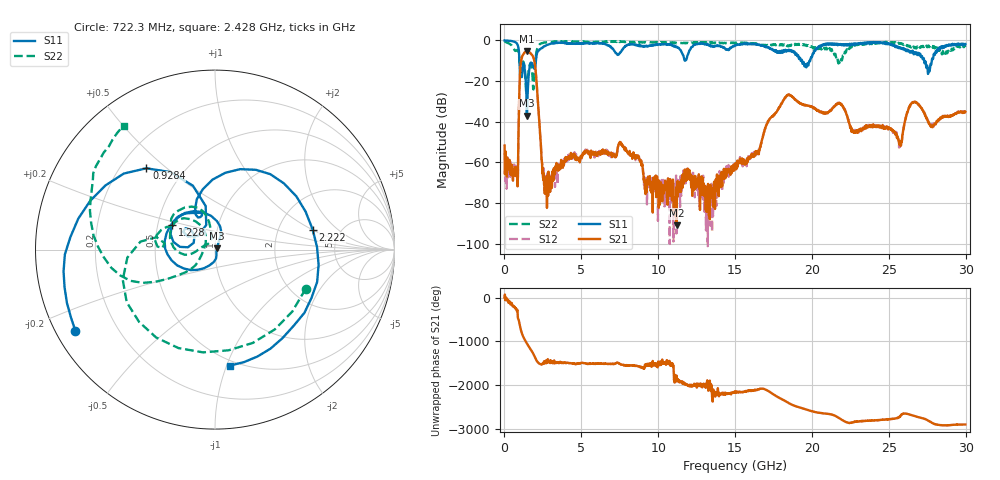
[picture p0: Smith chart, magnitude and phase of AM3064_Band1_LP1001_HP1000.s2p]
# Hz S DB R 50.0
!freq dBS11 angS11 dBS21 angS21 dBS12 angS12 dBS22 angS22
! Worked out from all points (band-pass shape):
!   1600 points, 10 MHz to 29.98 GHz, reference 50 ohm
!   highest |S21| = -5.26 dB at 1.472 GHz (marker M1); lowest = -91.1 dB at 11.2 GHz (marker M2)
!   |S21| within 3 dB of the highest: 1.133 GHz to 1.877 GHz (743.6 MHz wide, 49.4 % of centre)
!   lowest |S11| = -37.1 dB at 1.453 GHz (marker M3), VSWR 1.03, Z = 51.2 + j0.715 ohm
!   |S11| at or under -10 dB: 973.8 MHz to 2.042 GHz (1.068 GHz wide, 70.8 % of centre); 19.36 GHz to 19.84 GHz (479.9 MHz wide, 2.45 % of centre); 27.3 GHz to 27.79 GHz (493.8 MHz wide, 1.79 % of centre)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
!   |S22| runs from -26.0 to -0.3 dB; largest |S21 - S12| = 0.0059
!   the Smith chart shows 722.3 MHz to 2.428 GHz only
!   S11 on the Smith chart (normalised r, x): 722.3 MHz: 0.06, -0.27; 928.4 MHz: 0.31, +0.43; 1.228 GHz: 0.59, +0.17; 2.222 GHz: 3.15, +1.01; 2.428 GHz: 0.46, -1.03
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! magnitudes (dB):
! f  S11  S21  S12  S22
! 10 MHz  0.0  -51.8  -56.1  -0.3
! 722.3 MHz  -0.9  -63.7  -63.9  -5.2
! 928.4 MHz  -4.5  -39.4  -39.3  -6.2
! 1.228 GHz  -11.2  -6.8  -6.8  -10.5
! 1.453 GHz  -37.1  -5.3  -5.2  -24.5
! 1.472 GHz  -35.4  -5.3  -5.2  -22.9
! 1.922 GHz  -13.4  -9.3  -9.2  -19.0
! 2.222 GHz  -5.1  -34.9  -35.0  -2.5
! 2.428 GHz  -3.7  -59.2  -59.3  -1.4
! 2.69 GHz  -2.5  -70.3  -73.2  -1.0
! 5.015 GHz  -1.4  -56.7  -57.4  -0.7
! 7.582 GHz  -5.6  -50.6  -50.9  -0.7
! 10 GHz  -2.0  -76.6  -75.2  -0.9
! 11.2 GHz  -3.2  -91.1  -67.7  -1.2
! 15 GHz  -2.5  -62.3  -63.4  -1.4
! 18.36 GHz  -5.3  -27.1  -27.2  -2.6
! 19.99 GHz  -8.3  -32.7  -32.9  -3.0
! 25 GHz  -1.4  -43.2  -43.3  -1.1
! 25.75 GHz  -3.5  -50.6  -51.1  -1.6
! 26.63 GHz  -6.9  -30.3  -30.4  -3.1
! 27.56 GHz  -16.4  -39.8  -39.8  -2.7
! 29.98 GHz  -1.8  -35.1  -35.2  -3.2
